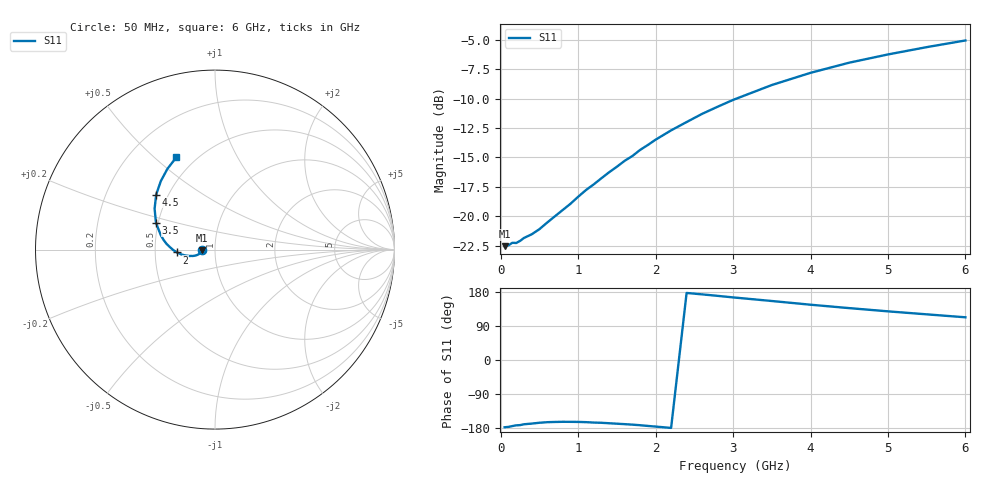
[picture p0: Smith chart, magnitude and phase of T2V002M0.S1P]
! SIEMENS Discrete & RF Semiconductors
! BAS70-04W
! Si Schottky Diode in SOT323
! IF = 2 mA
! S-Parameters:  November  1997
# GHz  S  MA  R  50
!  f  S11
! GHz  MAG  ANG
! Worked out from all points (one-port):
!   34 points, 50 MHz to 6 GHz, reference 50 ohm
!   lowest |S11| = -22.5 dB at 50 MHz (marker M1), VSWR 1.16, Z = 43.1 - j0.282 ohm
!   |S11| at or under -10 dB: start of sweep to 3.047 GHz
!   S11 on the Smith chart (normalised r, x): 50 MHz: 0.86, -0.01; 2 GHz: 0.65, -0.02; 3.5 GHz: 0.49, +0.17; 4.5 GHz: 0.43, +0.33; 6 GHz: 0.40, +0.59
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0.05  0.07471 -177.5
0.1  0.07533 -176.5
0.15  0.07722 -174.4
0.2  0.07707 -172.4
0.25  0.07869 -171.8
0.3  0.08095 -169.6
0.4  0.0839 -167.8
0.5  0.08822 -165.6
0.8  0.1064 -163.1
0.9  0.113 -163.2
1.1  0.1292 -164.0
1.2  0.1366 -165.1
1.3  0.1451 -165.7
1.6  0.172 -169.3
1.7  0.1803 -170.6
1.8  0.1914 -172.1
2  0.2115 -175.7
2.2  0.2316 -179.2
2.4  0.2512 176.9
2.6  0.2721 173.2
2.8  0.2917 169.3
3  0.3119 165.2
3.5  0.3607 155.7
4  0.4064 145.9
4.5  0.4488 136.9
5  0.4864 128.4
5.5  0.5223 120.5
6  0.5576 112.7
